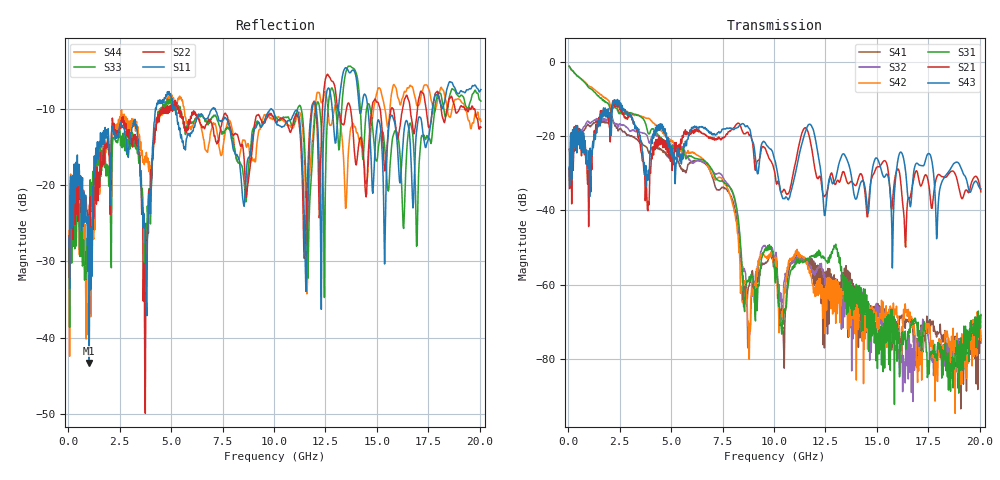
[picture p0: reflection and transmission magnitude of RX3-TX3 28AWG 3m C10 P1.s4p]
! FILE: O:\PROJECTS\SI-2007-05-003 3m Eyemax Qual\IL\RX3-TX3 28AWG 3m C10 P1.s4p
# MHZ S RI R 50.00
! FREQ  S11  S12  S13  S14
!  S21  S22  S23  S24
!  S31  S32  S33  S34
!  S41  S42  S43  S44
!  REAL  IMAG  REAL  IMAG  REAL  IMAG  REAL  IMAG
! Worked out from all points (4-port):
!   801 points, 50 MHz to 20.05 GHz, reference 50 ohm
!   strongest paths, dB at 50 MHz, 5.05 GHz, 10.05 GHz, 15.05 GHz, 20.05 GHz:
!     S43: -28.4, -25.5, -26.7, -26.4, -34.2
!     S21: -28.9, -29.2, -30.1, -28.3, -35.0
!     S31: -1.2, -23.0, -58.6, -73.7, -68.1
!     S42: -1.2, -21.6, -54.2, -69.0, -75.0
!     S32: -23.6, -22.9, -55.0, -65.8, -68.4
!     S41: -23.6, -26.9, -55.9, -65.2, -75.7
!   lowest |S11| = -43.3 dB at 1.025 GHz (marker M1), VSWR 1.01, Z = 49.3 + j0.126 ohm
!   |S11| at or under -10 dB: start of sweep to 4.248 GHz; 7.134 GHz to 11.87 GHz (4.731 GHz wide, 49.8 % of centre); 14.56 GHz to 17.7 GHz (3.137 GHz wide, 19.4 % of centre)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
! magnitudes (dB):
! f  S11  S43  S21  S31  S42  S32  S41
! 50 MHz  -26.9  -28.4  -28.9  -1.2  -1.2  -23.6  -23.6
! 1.025 GHz  -43.3  -23.9  -30.6  -7.0  -6.5  -16.4  -17.2
! 2.575 GHz  -12.0  -12.1  -13.3  -14.0  -13.5  -17.1  -18.1
! 7.45 GHz  -11.7  -18.6  -20.6  -32.1  -31.3  -30.4  -34.0
! 8.775 GHz  -16.4  -17.8  -19.5  -58.7  -72.1  -73.2  -60.5
! 9.525 GHz  -11.7  -21.5  -23.1  -51.1  -52.0  -49.7  -54.5
! 20.05 GHz  -7.5  -34.2  -35.0  -68.1  -75.0  -68.4  -75.7
